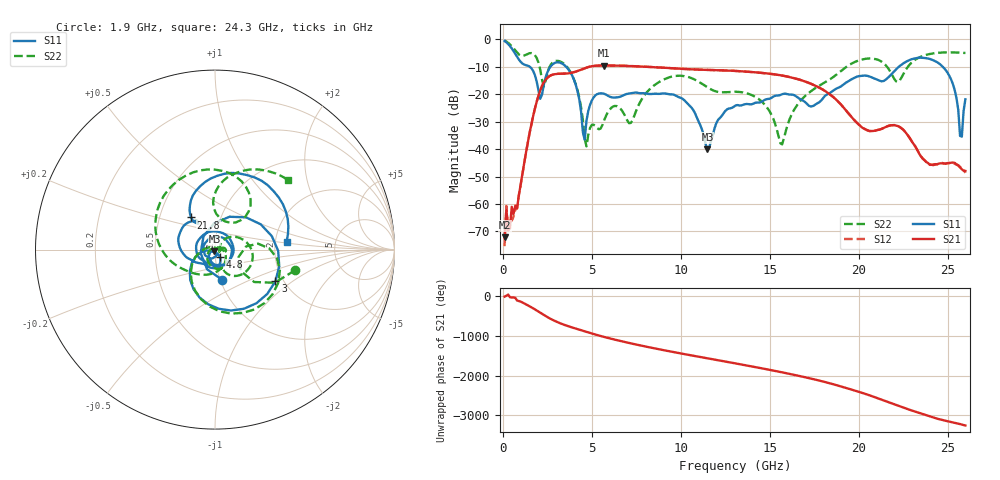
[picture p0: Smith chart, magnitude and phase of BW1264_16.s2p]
!Keysight Technologies,N5245B,MY57181159,A.13.60.06
!Date: Friday, December 18, 2020 23:52:44
!Correction: S11(Full 2 Port(1,2))
!S21(Full 2 Port(1,2))
!S12(Full 2 Port(1,2))
!S22(Full 2 Port(1,2))
!S2P File: Measurements: S11, S21, S12, S22:
# Hz S  dB  R 50
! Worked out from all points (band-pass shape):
!   260 points, 100 MHz to 26 GHz, reference 50 ohm
!   highest |S21| = -9.52 dB at 5.7 GHz (marker M1); lowest = -72.2 dB at 100 MHz (marker M2)
!   |S21| within 3 dB of the highest: 3.199 GHz to 15 GHz (11.8 GHz wide, 130 % of centre)
!   lowest |S11| = -40.1 dB at 11.5 GHz (marker M3), VSWR 1.02, Z = 49.7 - j0.943 ohm
!   |S11| at or under -10 dB: 1.519 GHz to 2.674 GHz (1.155 GHz wide, 55.1 % of centre); 3.559 GHz to 22.25 GHz (18.7 GHz wide, 145 % of centre); 24.73 GHz to end of sweep
!   |S22| runs from -39.0 to -0.4 dB; largest |S21 - S12| = 0.00055
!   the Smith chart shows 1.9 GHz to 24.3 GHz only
!   S11 on the Smith chart (normalised r, x): 1.9 GHz: 1.02, -0.35; 3 GHz: 1.82, -0.75; 4.8 GHz: 1.05, -0.09; 21.8 GHz: 0.72, +0.27; 24.3 GHz: 2.31, +0.24
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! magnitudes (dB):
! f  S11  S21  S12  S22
! 100 MHz  -0.6  -72.2  -75.4  -0.4
! 200 MHz  -1.1  -62.1  -60.7  -0.8
! 300 MHz  -1.7  -68.9  -69.8  -1.3
! 800 MHz  -6.3  -61.6  -61.6  -4.8
! 1.9 GHz  -15.3  -22.8  -22.8  -6.7
! 2.3 GHz  -16.7  -15.7  -15.7  -17.2
! 3 GHz  -8.4  -12.6  -12.6  -7.8
! 4 GHz  -14.7  -11.9  -11.9  -14.6
! 4.5 GHz  -33.9  -10.8  -10.8  -29.5
! 4.8 GHz  -26.1  -10.1  -10.1  -34.9
! 5.7 GHz  -19.8  -9.5  -9.5  -29.4
! 8.8 GHz  -19.9  -10.2  -10.2  -15.5
! 11.5 GHz  -40.1  -11.1  -11.1  -17.4
! 13.1 GHz  -24.0  -11.5  -11.5  -19.1
! 15.7 GHz  -20.0  -13.2  -13.2  -38.2
! 17.4 GHz  -24.4  -16.4  -16.4  -18.5
! 21.7 GHz  -13.7  -31.5  -31.5  -10.9
! 21.8 GHz  -13.0  -31.3  -31.3  -12.0
! 24.3 GHz  -7.9  -45.5  -45.7  -5.0
! 25.3 GHz  -16.3  -44.9  -45.0  -4.7
! 25.7 GHz  -35.2  -46.7  -46.4  -4.9
! 26 GHz  -21.8  -48.0  -48.6  -5.0
